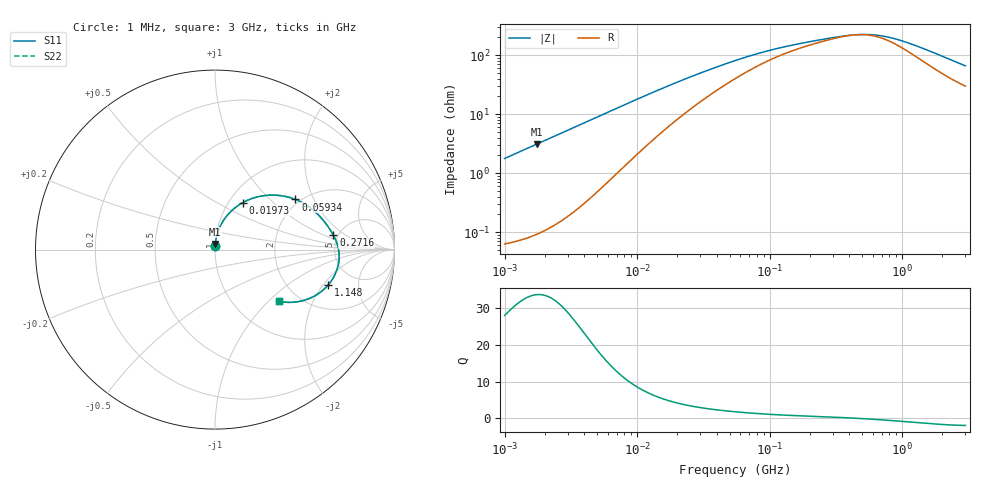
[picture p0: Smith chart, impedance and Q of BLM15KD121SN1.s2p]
! BLM15KD121SN1
# Hz S RI R 50
!Freq.(Hz) S11(Real) S11(Imag) S21(Real) S21(Imag) S12(Real) S12(Imag) S22(Real) S22(Imag)
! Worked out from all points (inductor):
!   401 points, 1 MHz to 3 GHz, reference 50 ohm
!   read as one part in series: L = 282 nH near 1.041 MHz
!   highest Q = 33.7 at 1.751 MHz (marker M1), where L = 282 nH
!   self-resonance near 449.7 MHz
!   S11 on the Smith chart (normalised r, x): 1 MHz: 1.00, +0.04; 19.73 MHz: 1.16, +0.67; 59.34 MHz: 1.88, +1.46; 271.6 MHz: 4.57, +1.31; 1.148 GHz: 3.18, -2.24; 3 GHz: 1.60, -1.17
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1000000  0.000943 0.0177  0.9991 -0.0177  0.9991 -0.0177  0.000943 0.0177
1751453  0.00188 0.0309  0.9981 -0.0309  0.9981 -0.0309  0.00188 0.0309
3823119  0.00739 0.0674  0.9926 -0.0674  0.9926 -0.0674  0.00739 0.0674
8179831  0.0335 0.1391  0.9665 -0.1391  0.9665 -0.1391  0.0335 0.1391
1.104425e7  0.0591 0.1792  0.9409 -0.1792  0.9409 -0.1792  0.0591 0.1792
1.461624e7  0.0964 0.22  0.9036 -0.22  0.9036 -0.22  0.0964 0.22
1.973457e7  0.1536 0.261  0.8464 -0.261  0.8464 -0.261  0.1536 0.261
3.320783e7  0.2883 0.3023  0.7117 -0.3023  0.7117 -0.3023  0.2883 0.3023
5.477226e7  0.4277 0.2866  0.5723 -0.2866  0.5723 -0.2866  0.4277 0.2866
5.933785e7  0.448 0.2794  0.552 -0.2794  0.552 -0.2794  0.448 0.2794
1.039275e8  0.5603 0.2088  0.4397 -0.2088  0.4397 -0.2088  0.5603 0.2088
2.094008e8  0.6391 0.1144  0.3609 -0.1144  0.3609 -0.1144  0.6391 0.1144
2.716345e8  0.6599 0.0797  0.3401 -0.0797  0.3401 -0.0797  0.6599 0.0797
3.817355e8  0.6816 0.0284  0.3184 -0.0284  0.3184 -0.0284  0.6816 0.0284
4.951867e8  0.6907 -0.018  0.3093 0.018  0.3093 0.018  0.6907 -0.018
6.296259e8  0.6897 -0.0666  0.3103 0.0666  0.3103 0.0666  0.6897 -0.0666
8.005644e8  0.6767 -0.1194  0.3233 0.1194  0.3233 0.1194  0.6767 -0.1194
1.147801e9  0.6287 -0.1992  0.3713 0.1992  0.3713 0.1992  0.6287 -0.1992
1.45942e9  0.5761 -0.2455  0.4239 0.2455  0.4239 0.2455  0.5761 -0.2455
1.893158e9  0.5031 -0.2807  0.4969 0.2807  0.4969 0.2807  0.5031 -0.2807
2.359433e9  0.4339 -0.2935  0.5661 0.2935  0.5661 0.2935  0.4339 -0.2935
3e9  0.3592 -0.2885  0.6408 0.2885  0.6408 0.2885  0.3592 -0.2885
